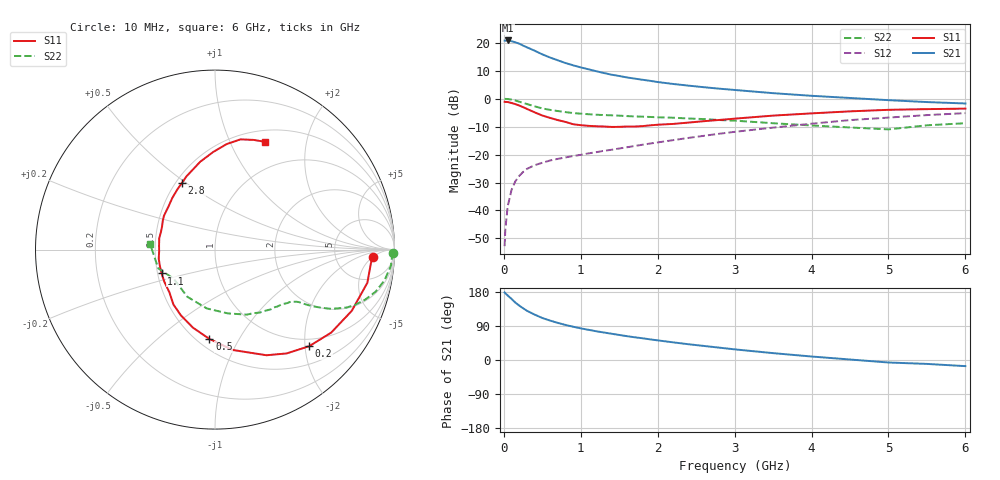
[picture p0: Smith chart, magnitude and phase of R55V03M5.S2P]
! SIEMENS Small Signal Semiconductors
! BFR183
! Si NPN RF Bipolar Junction Transistor in SOT23
! VCE = 5 V  IC = 3.5 mA
! Common Emitter S-Parameters:  May  1996
# GHz  S  MA  R  50
!  f  S11  S21  S12  S22
! GHz  MAG  ANG  MAG  ANG  MAG  ANG  MAG  ANG
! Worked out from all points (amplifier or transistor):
!   36 points, 10 MHz to 6 GHz, reference 50 ohm
!   highest |S21| = 20.8 dB at 50 MHz (marker M1)
!   |S21| within 3 dB of that: start of sweep to 345.4 MHz
!   unconditionally stable (mu >= 1): 1.199 GHz to 2.738 GHz
!   at 250 MHz: K = 0.32, MSG = 22.6 dB, |S12| = -26.2 dB
!   at 1.4 GHz: K = 1.05, MAG = 12.0 dB, |S12| = -18.3 dB
!   at 6 GHz: K = 0.88, MSG = 1.7 dB, |S12| = -5.2 dB
!   S11 on the Smith chart (normalised r, x): 10 MHz: 14, -5; 200 MHz: 0.84, -2.09; 500 MHz: 0.57, -0.76; 1.1 GHz: 0.53, -0.16; 2.8 GHz: 0.54, +0.48; 6 GHz: 0.64, +1.37
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0.01  0.8789 -2.6  10.87 178.2  0.0023 86.3  0.993 -1.0
0.02  0.872 -5.0  10.82 176.0  0.0047 91.2  0.9874 -2.1
0.05  0.8687 -12.3  10.95 170.3  0.0118 82.5  0.9844 -5.3
0.1  0.8349 -24.1  10.59 161.2  0.0233 77.5  0.9591 -10.4
0.15  0.7958 -35.5  10.13 151.4  0.0333 71.9  0.9249 -14.7
0.2  0.7518 -45.7  9.602 143.6  0.0416 66.6  0.8812 -18.5
0.25  0.7028 -55.4  8.871 136.5  0.0488 63.2  0.8382 -21.6
0.3  0.6549 -64.0  8.253 130.0  0.0553 59.9  0.8004 -23.8
0.4  0.5679 -80.0  7.194 119.8  0.0645 55.2  0.7274 -27.0
0.5  0.4986 -93.6  6.18 110.9  0.0712 53.1  0.6679 -28.9
0.6  0.4522 -105.7  5.43 104.1  0.0782 51.6  0.6292 -30.1
0.7  0.4131 -117.3  4.846 98.0  0.0836 51.0  0.5998 -30.9
0.8  0.3836 -127.2  4.331 92.6  0.0887 50.8  0.5735 -31.5
1.1  0.3258 -155.9  3.338 79.7  0.1048 52.9  0.5254 -33.6
1.4  0.3114 -178.2  2.677 69.3  0.1216 54.3  0.5024 -36.3
1.6  0.3171 168.3  2.389 62.9  0.1348 55.1  0.487 -38.4
2.2  0.3525 137.6  1.828 46.6  0.1808 56.0  0.4553 -47.0
2.8  0.4151 116.2  1.506 32.6  0.2353 53.6  0.4139 -58.8
3.5  0.4966 99.5  1.251 18.1  0.3028 47.5  0.3627 -78.6
4.5  0.5915 83.7  1.026 1.3  0.4128 36.1  0.3047 -120.4
5.5  0.6482 70.5  0.867 -10.3  0.5071 23.1  0.333 -161.7
6  0.6622 65.0  0.818 -16.2  0.5503 14.7  0.3631 175.0
